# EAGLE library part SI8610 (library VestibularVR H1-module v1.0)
DGTL ISO 3750VRMS 1CH GP 8SOIC
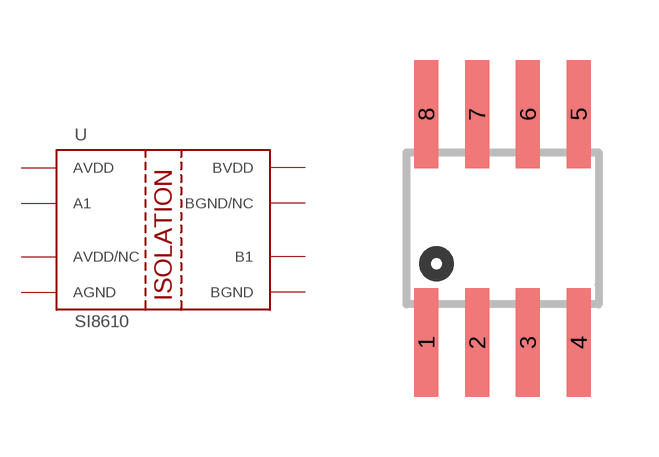
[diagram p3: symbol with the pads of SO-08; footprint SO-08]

Designator prefix -

## SI8610  [SO-08]
1  AVDD
2  A1
3  AVDD/NC
4  AGND
5  BGND
6  B1
7  BGND/NC
8  BVDD

## Footprint SO-08 (pad centres in mm)
smd 0.6 x 2.708: 1 -1.905,-2.854; 2 -0.635,-2.854; 3 0.635,-2.854; 4 1.905,-2.854; 5 1.905,2.854; 6 0.635,2.854; 7 -0.635,2.854; 8 -1.905,2.854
